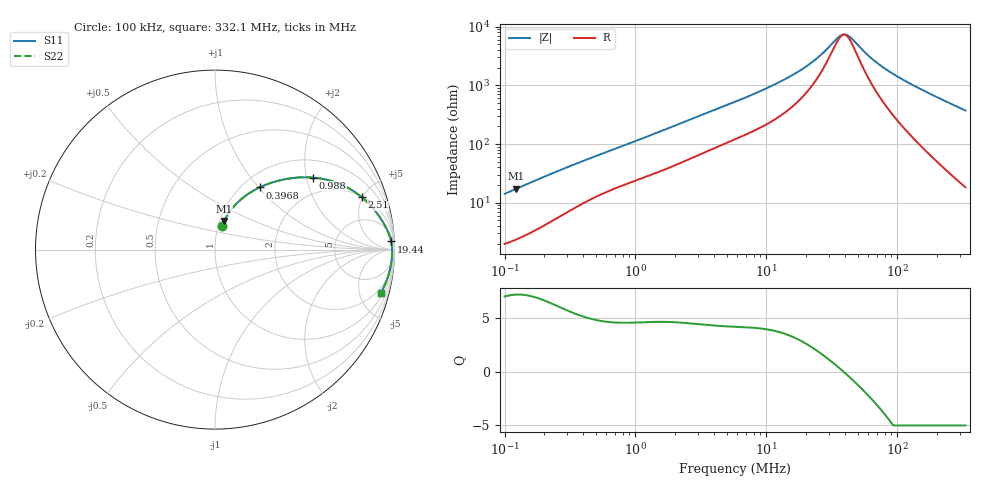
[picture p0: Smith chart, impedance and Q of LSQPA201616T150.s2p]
! LSQPA201616T150  S-PARAMETER MODEL  ( General Type )
! Model Generated by TAIYO YUDEN Corporation (http://www.ty-top.com)
! Version 2.0
! TAIYO YUDEN Control No. 100810NF25SB-FKC
! Copyright(c) 2007 TAIYO YUDEN CO.,LTD. All Rights Reserved.
! Product Description (link to TY-COMPAS)
! https://ds.yuden.co.jp/TYCOMPAS/or/detail?pn=LSQPA201616T150K&u=M
! Products Name : Inductors
! Characteristics :
!  Inductance : 15 uH , SRF(min) : 28 MHz , DC Resistance(max) : 1.56 Ohm
!  Rated Current : Saturation :300 mA , Temp Rise : 300 mA (40 degC)
!  Case Size : 2.0 x 1.6 / 0.079 x 0.063 [mm/inch] , Thickness : 1.6 / 0.063 [mm/inch]
!  (Conditions: Temperature = 25 degC , DC Bias Current/Voltage = 0A / 0V)
! External Node Assignments :
!  1  o---GGG---o  2
! GND o---------o GND
! Frequency Range : 0.1MHz  -  332.076389MHz  [ 402 STEP ]
# MHz S RI R 50
! Freq[MHz].  S11 Real  S11 Imag  S21 Real  S21 Imag  S12 Real  S12 Imag  S22 Real  S22 Imag
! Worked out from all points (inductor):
!   401 points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, 100 kHz to 332.1 MHz, reference 50 ohm
!   read as one part in series: L = 22.2 uH near 104.1 kHz
!   highest Q = 7.23 at 122.5 kHz (marker M1), where L = 22.3 uH
!   self-resonance near 39.12 MHz
!   S11 on the Smith chart (normalised r, x): 100 kHz: 1.04, +0.28; 396.8 kHz: 1.19, +1.01; 988 kHz: 1.47, +2.18; 2.51 MHz: 2.08, +4.92; 19.44 MHz: 15, +37; 332.1 MHz: 1.37, -7.46
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0.1  0.0378 0.1326  0.9622 -0.1326  0.9622 -0.1326  0.0378 0.1326
0.12247  0.0498 0.1591  0.9502 -0.1591  0.9502 -0.1591  0.0498 0.1591
0.220455  0.1167 0.2531  0.8833 -0.2531  0.8833 -0.2531  0.1167 0.2531
0.388873  0.2428 0.3436  0.7572 -0.3436  0.7572 -0.3436  0.2428 0.3436
0.396835  0.2484 0.3463  0.7516 -0.3463  0.7516 -0.3463  0.2484 0.3463
0.645483  0.3977 0.3936  0.6023 -0.3936  0.6023 -0.3936  0.3977 0.3936
0.987984  0.5442 0.4014  0.4558 -0.4014  0.4558 -0.4014  0.5442 0.4014
1.512219  0.687 0.3691  0.313 -0.3691  0.313 -0.3691  0.687 0.3691
2.510106  0.8174 0.2919  0.1826 -0.2919  0.1826 -0.2919  0.8174 0.2919
5.762607  0.9285 0.1652  0.0715 -0.1652  0.0715 -0.1652  0.9285 0.1652
11.7146  0.9687 0.0871  0.0313 -0.0871  0.0313 -0.0871  0.9687 0.0871
19.44486  0.981 0.0456  0.019 -0.0456  0.019 -0.0456  0.981 0.0456
22.4092  0.9829 0.0356  0.0171 -0.0356  0.0171 -0.0356  0.9829 0.0356
26.89393  0.9847 0.0235  0.0153 -0.0235  0.0153 -0.0235  0.9847 0.0235
35.71886  0.9863 0.00562  0.0137 -0.00562  0.0137 -0.00562  0.9863 0.00562
37.95831  0.9865 0.00187  0.0135 -0.00187  0.0135 -0.00187  0.9865 0.00187
40.33816  0.9867 -0.00189  0.0133 0.00189  0.0133 0.00189  0.9867 -0.00189
44.64076  0.9868 -0.00819  0.0132 0.00819  0.0132 0.00819  0.9868 -0.00819
64.2965  0.9863 -0.0321  0.0137 0.0321  0.0137 0.0321  0.9863 -0.0321
87.14324  0.9845 -0.0552  0.0155 0.0552  0.0155 0.0552  0.9845 -0.0552
153.7165  0.9745 -0.1129  0.0255 0.1129  0.0255 0.1129  0.9745 -0.1129
332.0764  0.9228 -0.2435  0.0772 0.2435  0.0772 0.2435  0.9228 -0.2435
